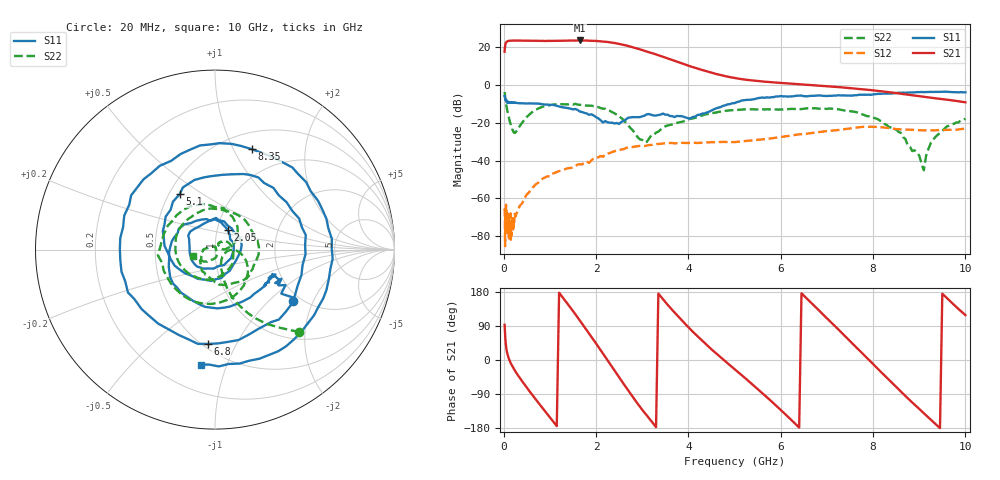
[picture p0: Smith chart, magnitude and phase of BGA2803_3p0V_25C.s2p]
#  HZ  S  RI  R  50.0000
! Rohde & Schwarz ZVA/B
! Temperature 25C
! Device number 102
! Measured Vcc 3.000000
! Measured Icc 0.005700
! DeltaGain  -0.131549  3dBBWHighMHz 2746.04  3dBBWLowMHz 28.89
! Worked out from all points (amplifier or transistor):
!   242 points, 20 MHz to 10 GHz, reference 50 ohm
!   highest |S21| = 23.7 dB at 1.65 GHz (marker M1)
!   |S21| within 3 dB of that: 30.53 MHz to 2.707 GHz (2.676 GHz wide, 196 % of centre)
!   unconditionally stable (mu >= 1): start of sweep to end of sweep
!   at 220 MHz: K = 107.27, MAG = 24.1 dB, |S12| = -71.3 dB
!   at 4 GHz: K = 5.08, MAG = 10.5 dB, |S12| = -30.6 dB
!   at 10 GHz: K = 11.61, MAG = -6.7 dB, |S12| = -23.0 dB
!   S11 on the Smith chart (normalised r, x): 20 MHz: 1.82, -1.41; 2.05 GHz: 1.12, +0.25; 5.1 GHz: 0.57, +0.40; 6.8 GHz: 0.53, -0.77; 8.35 GHz: 0.69, +1.19; 10 GHz: 0.37, -0.82
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2e7  0.433 -0.284  -0.3802 7.653  0.000457 -0.000172  0.4702 -0.4597
6e7  0.3629 -0.1724  12.18 6.573  -0.00035 -0.000353  0.0965 -0.2671
1.3e8  0.3125 -0.1547  14.97 -0.5417  9.27e-05 -0.000141  0.0348 -0.1063
3.5e8  0.2181 -0.2466  10.21 -11.17  -0.000641 -1.34e-05  0.0816 -0.00229
6.5e8  0.0146 -0.3275  -1.792 -14.88  -0.00111 0.00174  0.1817 -0.0943
9.5e8  -0.1903 -0.2393  -11.9 -8.804  0.00117 0.00368  0.068 -0.2804
1.2e9  -0.2578 -0.0915  -14.91 0.6164  0.00402 0.00341  -0.1452 -0.2762
1.4e9  -0.2402 0.0476  -12.47 8.565  0.00605 0.0018  -0.2668 -0.1532
1.65e9  -0.134 0.148  -3.691 14.78  0.00795 -0.00102  -0.2954 0.0545
1.7e9  -0.1087 0.1594  -1.441 15.1  0.00776 -0.00166  -0.283 0.0908
2.05e9  0.0705 0.1111  11.98 8.363  0.00865 -0.00867  -0.0637 0.2538
2.3e9  0.0984 -0.021  13.42 -2.318  0.00476 -0.0152  0.0965 0.1844
2.65e9  -0.0637 -0.1063  3.503 -10.71  -0.0099 -0.0192  0.0965 0.0238
3e9  -0.1433 0.0381  -5.592 -6.366  -0.0238 -0.00685  0.0333 0.0116
3.35e9  -0.0414 0.1553  -6.161 0.5199  -0.0251 0.0112  0.0404 0.0425
4.15e9  0.0584 -0.1347  1.054 2.652  0.0132 0.0265  0.0663 -0.1187
5.05e9  -0.2346 0.2665  1.315 -0.7345  0.0284 -0.0135  -0.2203 -0.00505
5.1e9  -0.1964 0.3091  1.213 -0.8335  0.0276 -0.0158  -0.2206 0.0204
6.7e9  0.0796 -0.513  -0.8305 0.5498  -0.054 0.00533  0.2433 -0.00732
6.8e9  -0.0414 -0.5256  -0.6812 0.6951  -0.0542 0.0157  0.2358 -0.0448
8.35e9  0.2071 0.5589  0.3927 -0.5183  0.0705 -0.0179  -0.0719 -0.0268
1e10  -0.0775 -0.6406  -0.1673 0.3087  -0.0678 -0.0206  -0.1238 -0.0368
